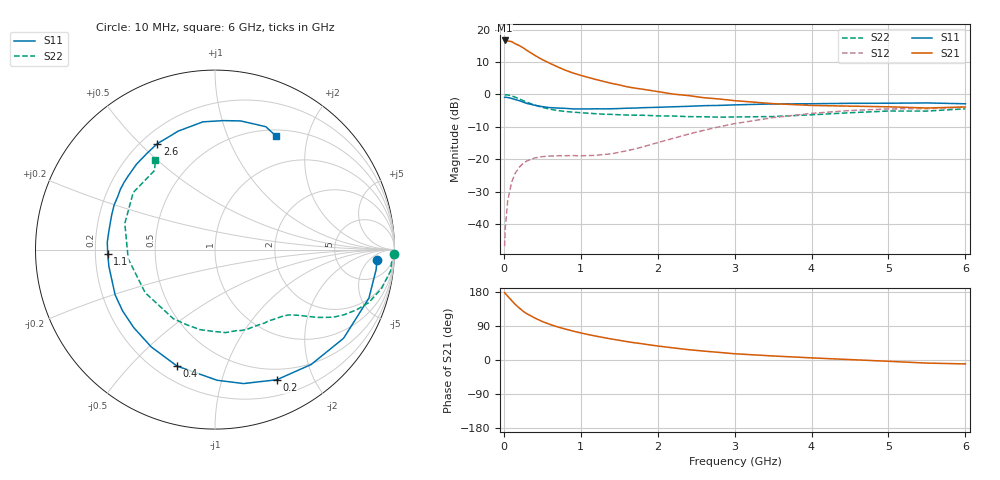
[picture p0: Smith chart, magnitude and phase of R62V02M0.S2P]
! SIEMENS Small Signal Semiconductors
! BFR193
! Si NPN RF Bipolar Junction Transistor in SOT23
! VCE = 2 V  IC = 2 mA
! Common Emitter S-Parameters:  May  1996
# GHz  S  MA  R  50
!  f  S11  S21  S12  S22
! GHz  MAG  ANG  MAG  ANG  MAG  ANG  MAG  ANG
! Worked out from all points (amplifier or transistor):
!   36 points, 10 MHz to 6 GHz, reference 50 ohm
!   highest |S21| = 16.6 dB at 10 MHz (marker M1)
!   |S21| within 3 dB of that: start of sweep to 296.4 MHz
!   unconditionally stable (mu >= 1): 1.151 GHz to 2.053 GHz
!   at 250 MHz: K = 0.24, MSG = 17.8 dB, |S12| = -21.2 dB
!   at 1.4 GHz: K = 1.13, MAG = 8.7 dB, |S12| = -18.3 dB
!   at 6 GHz: K = 1.00, MSG = 0.0 dB, |S12| = -3.9 dB
!   S11 on the Smith chart (normalised r, x): 10 MHz: 15, -9; 200 MHz: 0.37, -1.52; 400 MHz: 0.28, -0.69; 1.1 GHz: 0.25, -0.02; 2.6 GHz: 0.26, +0.56; 6 GHz: 0.57, +1.51
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0.01  0.9046 -3.5  6.796 178.0  0.0046 89.0  0.9978 -1.3
0.02  0.9045 -7.1  6.734 175.2  0.0092 87.0  0.9881 -2.7
0.05  0.8991 -17.5  6.67 168.4  0.0229 80.7  0.9856 -6.9
0.1  0.8702 -34.6  6.523 157.3  0.0441 71.7  0.9523 -13.2
0.15  0.8347 -50.1  6.039 146.4  0.0617 63.2  0.9063 -19.0
0.2  0.8027 -64.6  5.668 137.3  0.0756 56.7  0.8567 -23.1
0.25  0.7631 -78.0  5.251 128.8  0.0866 50.7  0.8037 -26.9
0.3  0.728 -89.1  4.779 122.0  0.0945 46.0  0.7583 -29.8
0.4  0.6826 -108.0  4.025 111.2  0.1051 39.4  0.6885 -33.3
0.5  0.6482 -123.3  3.444 101.5  0.1101 35.1  0.6341 -35.9
0.6  0.6274 -136.3  3.018 93.9  0.1125 32.7  0.5935 -38.1
0.7  0.618 -146.4  2.658 87.2  0.1133 31.8  0.5665 -40.0
0.9  0.5992 -163.5  2.141 76.3  0.1144 32.4  0.5347 -43.6
1.1  0.5983 -177.7  1.828 67.0  0.1144 36.6  0.5136 -48.3
1.4  0.6022 165.5  1.483 55.3  0.122 46.4  0.4939 -55.9
1.6  0.6145 156.0  1.314 48.5  0.1362 52.8  0.4823 -61.8
2.2  0.6464 132.5  1.014 32.0  0.2105 62.1  0.4661 -82.9
2.6  0.6722 118.6  0.891 23.5  0.2806 60.1  0.4536 -100.6
3.5  0.715 95.4  0.722 10.6  0.44 44.6  0.4571 -148.2
4.5  0.7309 78.8  0.661 1.1  0.5661 23.8  0.5232 163.8
5.5  0.7409 67.5  0.619 -8.2  0.6032 4.9  0.5549 127.4
6  0.7188 62.0  0.642 -10.3  0.6359 -0.3  0.6014 123.5
